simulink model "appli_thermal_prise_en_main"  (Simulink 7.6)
settings: Solver=ode15s  StartTime=0.0  StopTime=2000  RelTol=1e-3
StopFcn:
  | close all
  | load temp.mat
  | plot(x(1,:),x(2,:),x(1,:),x(3,:))
  | title('Réponse d''une masse thermique à un échelon de température')
  | xlabel('temps')
  | gtext('température de la masse thermique')
  | gtext('échelon de température d''entrée')
  | grid
libraries: fl_lib x8, nesl_utility x4

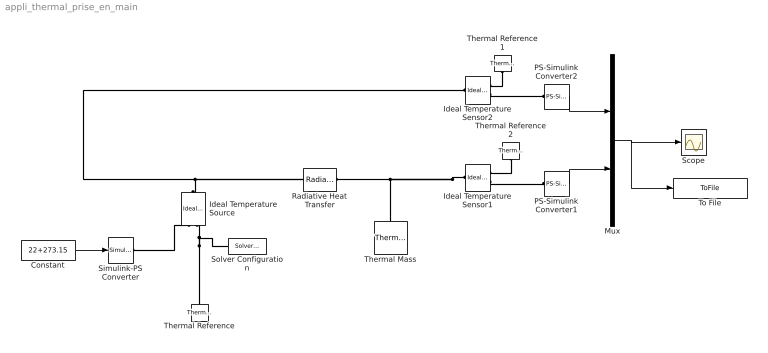
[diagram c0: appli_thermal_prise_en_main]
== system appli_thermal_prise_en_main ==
  Constant : Constant  Value=22+273.15
  Ideal Temperature Sensor1 : fl_lib/Thermal/Thermal Sensors/Ideal Temperature Sensor  DialogController=NetworkEngine.DynNeDlgSource  SystemSampleTime=-1  Qs_Log=off  Ts_Log=off  LocalVarNames=|Qs|Ts  LocalVarDescs=|Qs|Ts  LocalVarLogging=[0 0]
  Ideal Temperature Sensor2 : fl_lib/Thermal/Thermal Sensors/Ideal Temperature Sensor  DialogController=NetworkEngine.DynNeDlgSource  SystemSampleTime=-1  Qs_Log=off  Ts_Log=off  LocalVarNames=|Qs|Ts  LocalVarDescs=|Qs|Ts  LocalVarLogging=[0 0]
  Ideal Temperature Source : fl_lib/Thermal/Thermal Sources/Ideal Temperature Source  DialogController=NetworkEngine.DynNeDlgSource  SystemSampleTime=-1  Q_Log=off  T_Log=off  LocalVarNames=|Q|T  LocalVarDescs=|Q|T  LocalVarLogging=[0 0]
  Mux : Mux  Inputs=2
  PS-Simulink Converter1 : nesl_utility/PS-Simulink Converter  DialogController=NetworkEngine.DynNeUtilDlgSource  SystemSampleTime=-1  PhysicalDomain=network_engine_domain  LeftPortType=input  RightPortType=output  SubClassName=ps_output  Unit=1  AffineConversion=off
  PS-Simulink Converter2 : nesl_utility/PS-Simulink Converter  DialogController=NetworkEngine.DynNeUtilDlgSource  SystemSampleTime=-1  PhysicalDomain=network_engine_domain  LeftPortType=input  RightPortType=output  SubClassName=ps_output  Unit=1  AffineConversion=off
  Radiative Heat Transfer : fl_lib/Thermal/Thermal Elements/Radiative Heat Transfer  DialogController=NetworkEngine.DynNeDlgSource  SystemSampleTime=-1  area=1 m^2  rad_tr_coeff=4e-08 W/(m^2*K^4)  Q_Log=off  LocalVarNames=|Q  LocalVarDescs=|Q  LocalVarLogging=0
  Scope : Scope
  Simulink-PS Converter : nesl_utility/Simulink-PS Converter  DialogController=NetworkEngine.DynNeUtilDlgSource  SystemSampleTime=-1  PhysicalDomain=network_engine_domain  LeftPortType=input  RightPortType=output  SubClassName=ps_input  Unit=1  AffineConversion=off  InputFilterTimeConstant=.001  UdotUserProvided=0
  Solver Configuration : nesl_utility/Solver Configuration  DialogController=NetworkEngine.DynNeUtilDlgSource  SystemSampleTime=-1  PhysicalDomain=network_engine_domain  LeftPortType=input  RightPortType=generic  SubClassName=solver  Accelerate=off  Profile=off  ResidualTolerance=1e-9  MaxNonlinIter=12  MaxModeIter=2  DoFixedCost=off  UseLocalSampling=off  DoDC=on  LinearAlgebra=Full  LocalSolverSampleTime=.001  LocalSolverChoice=NE_BACKWARD_EULER_ADVANCER  UseLocalSolver=off
  Thermal Mass : fl_lib/Thermal/Thermal Elements/Thermal Mass  DialogController=NetworkEngine.DynNeDlgSource  SystemSampleTime=-1  mass=1 kg  sp_heat=447 J/kg/K  init_temp=0 C  Q_Log=off  LocalVarNames=|Q  LocalVarDescs=|Q  LocalVarLogging=0
  Thermal Reference : fl_lib/Thermal/Thermal Elements/Thermal Reference  DialogController=NetworkEngine.DynNeDlgSource  SystemSampleTime=-1  Q_Log=off  LocalVarNames=|Q  LocalVarDescs=|Q  LocalVarLogging=0
  Thermal Reference1 : fl_lib/Thermal/Thermal Elements/Thermal Reference  DialogController=NetworkEngine.DynNeDlgSource  SystemSampleTime=-1  Q_Log=off  LocalVarNames=|Q  LocalVarDescs=|Q  LocalVarLogging=0
  Thermal Reference2 : fl_lib/Thermal/Thermal Elements/Thermal Reference  DialogController=NetworkEngine.DynNeDlgSource  SystemSampleTime=-1  Q_Log=off  LocalVarNames=|Q  LocalVarDescs=|Q  LocalVarLogging=0
  To File : ToFile  Filename=temp.mat  MatrixName=x
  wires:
  Mux/1 -> Scope/1, To File/1
  PS-Simulink Converter2/1 -> Mux/1
  PS-Simulink Converter1/1 -> Mux/2
  Constant/1 -> Simulink-PS Converter/1
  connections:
  Ideal Temperature Sensor1/RConn2 -- PS-Simulink Converter1/LConn1
  Thermal Reference2/LConn1 -- Ideal Temperature Sensor1/RConn1
  Simulink-PS Converter/RConn1 -- Ideal Temperature Source/RConn1
  Ideal Temperature Source/RConn2 -- Thermal Reference/LConn1 -- Solver Configuration/RConn1
  Ideal Temperature Source/LConn1 -- Ideal Temperature Sensor2/LConn1 -- Radiative Heat Transfer/LConn1
  Ideal Temperature Sensor1/LConn1 -- Thermal Mass/LConn1 -- Radiative Heat Transfer/RConn1
  Thermal Reference1/LConn1 -- Ideal Temperature Sensor2/RConn1
  Ideal Temperature Sensor2/RConn2 -- PS-Simulink Converter2/LConn1
